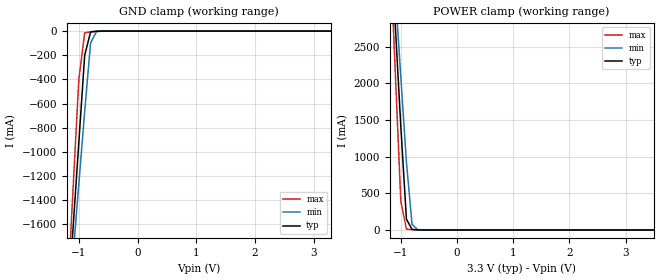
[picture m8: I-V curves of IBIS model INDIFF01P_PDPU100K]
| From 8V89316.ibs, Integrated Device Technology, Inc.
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[Model]   INDIFF01P_PDPU100K
Model_type   Input
Polarity   Non-Inverting
Vinl = 0.8V
Vinh = 2.0V
|   typ   min   max
C_comp   2pF   1.5pF   2.5pF
|   typ   min   max
[Voltage range]   3.3V   3.135V   3.465V
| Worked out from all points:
|   GND clamp passes 1 mA (typ) near -0.68 V on its own axis
|   POWER clamp passes 1 mA (typ) near -0.64 V on its own axis
[GND_clamp]
|Voltage   I (typ)   I (min)   I (max)
-3.3V     -17.55A    -15.11A    -21.66A
-1.2V     -2.37A     -2.47A     -2.252A
-1.1V     -1.646A    -1.868A    -1.326A
-1V       -923.2mA   -1.267A    -401.1mA
-900mV    -200.8mA   -666.1mA   -14.91mA
-800mV    -7.668mA   -98.79mA   -5.444mA
-700mV    -1.231mA   -4.677mA   -1.652mA
3.3V      32.92uA    30.78uA    35.01uA
[Power_clamp]
|Voltage   I (typ)   I (min)   I (max)
-3.3V     33.64A     28.92A     41.58A
-1.2V     4.209A     4.413A     3.966A
-1.1V     2.811A     3.249A     2.179A
-1V       1.414A     2.086A     391.8mA
-900mV    147.2mA    923.6mA    11.36mA
-800mV    6.929mA    74.46mA    4.764mA
-700mV    1.686mA    4.432mA    2.103mA
3.5V      -1.998uA   -4.445uA   -371.3nA
